| IBIS file stm32wba63_a65_vqfpn68_smps_usb.ibs
[IBIS ver] 4.2
[File name] stm32wba63_a65_vqfpn68_smps_usb.ibs
[File Rev] 2.0
[Date] 17-02-2025
[Source] Data Created at STMicroelectronics
[Notes]  File originated from ELDO simulations.
[Disclaimer]  This information is for modeling purpose only and is
   not guaranted. The information is subject to change without
   notice.
[Copyright] Copyright 2025 STMicroelectronics Inc.
|   Component stm32wba63_a65_vqfpn68_smps_usb
[Component] stm32wba63_a65_vqfpn68_smps_usb
[Manufacturer] STMicroelectronics
[Package]
| variable   typ   min   max
R_pkg  0  NA  NA
L_pkg  0  NA  NA
C_pkg  0  NA  NA
[Pin]   signal_name   model_name
0  VSS  gnd
1  VSSSMPS  nc
2  VDDSMPS  nc
3  VLXSMPS  nc
4  PB12  io8_ft_100m
5  PB11  io8_ft_100m_i2c
6  PA8  io8_ft_100m
7  PA7  io8_ft_100m_i2c_v33
8  PA6  io8_ft_100m_i2c
9  VREFP  nc
10  VDDA  nc
11  PA5  io8_ft_100m
12  PA4  io8_ft_100m_v33
13  PA3  io8_ft_100m
14  PB10  io8_ft_100m_i2c
15  PA2  io8_ft_100m_v33
16  VDD  power
17  PA1  io8_ft_100m
18  PA0  io8_ft_100m
19  PB9  io8_ft_100m
20  VDDUSB  power
21  PD9  io8_ft_100m
22  PD8  io8_ft_100m
23  PD7  io8_ft_100m
24  PD6  io8_ft_100m
25  PD5  io8_ft_100m
26  PB8  io8_ft_100m
27  VDD  power
28  PC15-OSC32_OUT  io_ft_tamp
29  PC14-OSC32_IN  io_ft_tamp
30  PC13  io8_ft_100m_v33
31  VDD  power
32  PB4  io8_ft_100m
33  PE3  io8_ft_100m_hslv
34  PE2  io8_ft_100m_hslv
35  PE1  io8_ft_100m_hslv
36  PE0  io8_ft_100m_hslv
37  PD14  io8_ft_100m_hslv
38  VDD  power
39  PB3  io8_ft_100m_i2c
40  PA15  io8_ft_100m_i2c
41  PA14  io8_ft_100m_v33
42  PA13  io8_ft_100m
43  PA12  io8_ft_100m
44  PA11  io8_ft_100m
45  PB2  io8_ft_100m_i2c_v33
46  PB1  io8_ft_100m_i2c
47  PB0  io8_ft_100m
48  PB15  io8_ft_100m
49  PH3-BOOT0  io8_ft_100m_v33
50  VDD  power
51  NRST  ioreset_v33
52  RF  nc
53  VDDHPA  nc
54  VDDANA  nc
55  VDDRF  nc
56  OSC_OUT  nc
57  OSC_IN  nc
58  VDDRFPA  nc
59  VDD-59  power
60  VDD11  nc
61  PC5  io8_ft_100m
62  PC4  io8_ft_100m
63  PC3  io8_ft_100m
64  PA10  io8_ft_100m
65  PA9  io8_ft_100m
66  PB14  io8_ft_100m_i2c
67  PB13  io8_ft_100m_i2c
68  VDD-68  power
[Package Model]   4b0-vqfn-8x8-68-240827
[Pin Mapping]   pulldown_ref   pullup_ref   | Comment
0  gndio  nc
1  nc  nc
2  nc  nc
3  nc  nc
4  gndio  vddio
5  gndio  vddio
6  gndio  vddio
7  gndio  vddio
8  gndio  vddio
9  nc  nc
10  nc  nc
11  gndio  vddio
12  gndio  vddio
13  gndio  vddio
14  gndio  vddio
15  gndio  vddio
16  nc  vddio
17  gndio  vddio
18  gndio  vddio
19  gndio  vddio
20  nc  vddusb
21  gndio  vddio  | Depending on IO usage
| 21  gndio  vddusb  | Depending on IO usage
22  gndio  vddio  | Depending on IO usage
| 22  gndio  vddusb  | Depending on IO usage
23  gndio  vddio
24  gndio  vddio
25  gndio  vddio
26  gndio  vddio
27  nc  vddio
28  gndio  vddio
29  gndio  vddio
30  gndio  vddio
31  nc  vddio
32  gndio  vddio
33  gndio  vddio
34  gndio  vddio
35  gndio  vddio
36  gndio  vddio
37  gndio  vddio
38  nc  vddio
39  gndio  vddio
40  gndio  vddio
41  gndio  vddio
42  gndio  vddio
43  gndio  vddio
44  gndio  vddio
45  gndio  vddio
46  gndio  vddio
47  gndio  vddio
48  gndio  vddio
49  gndio  vddio
50  nc  vddio
51  gndio  vddio
52  nc  nc
53  nc  nc
54  nc  nc
55  nc  nc
56  nc  nc
57  nc  nc
58  nc  nc
59  nc  vddio
60  nc  nc
61  gndio  vddio
62  gndio  vddio
63  gndio  vddio
64  gndio  vddio
65  gndio  vddio
66  gndio  vddio
67  gndio  vddio
68  nc  vddio
|[Diff Pin]  inv_pin  vdiff  tdelay_typ  tdelay_min  tdelay_max
|24  23  NA  NA  NA  NA
[Model Selector] io8_ft_100m
io8_ft_100m_ls_1v2  "GPIO 100MHz - 5V tolerant - low speed - 1.2V range"
io8_ft_100m_ls_1v8  "GPIO 100MHz - 5V tolerant - low speed - 1.8V range"
io8_ft_100m_ls_3v3  "GPIO 100MHz - 5V tolerant - low speed - 3.3V range"
io8_ft_100m_ms_1v2  "GPIO 100MHz - 5V tolerant - med speed - 1.2V range"
io8_ft_100m_ms_1v8  "GPIO 100MHz - 5V tolerant - med speed - 1.8V range"
io8_ft_100m_ms_3v3  "GPIO 100MHz - 5V tolerant - med speed - 3.3V range"
io8_ft_100m_fs_1v2  "GPIO 100MHz - 5V tolerant - fast speed - 1.2V range"
io8_ft_100m_fs_1v8  "GPIO 100MHz - 5V tolerant - fast speed - 1.8V range"
io8_ft_100m_fs_3v3  "GPIO 100MHz - 5V tolerant - fast speed - 3.3V range"
io8_ft_100m_hs_1v2  "GPIO 100MHz - 5V tolerant - high speed - 1.2V range"
io8_ft_100m_hs_1v8  "GPIO 100MHz - 5V tolerant - high speed - 1.8V range"
io8_ft_100m_hs_3v3  "GPIO 100MHz - 5V tolerant - high speed - 3.3V range"
[Model Selector] io8_ft_100m_hslv
io8_ft_100m_ls_1v2  "GPIO 100MHz - 5V tolerant - low speed - 1.2V range"
io8_ft_100m_ls_1v8  "GPIO 100MHz - 5V tolerant - low speed - 1.8V range"
io8_ft_100m_ls_3v3  "GPIO 100MHz - 5V tolerant - low speed - 3.3V range"
io8_ft_100m_ms_1v2  "GPIO 100MHz - 5V tolerant - med speed - 1.2V range"
io8_ft_100m_ms_1v8  "GPIO 100MHz - 5V tolerant - med speed - 1.8V range"
io8_ft_100m_ms_3v3  "GPIO 100MHz - 5V tolerant - med speed - 3.3V range"
io8_ft_100m_fs_1v2  "GPIO 100MHz - 5V tolerant - fast speed - 1.2V range"
io8_ft_100m_fs_1v8  "GPIO 100MHz - 5V tolerant - fast speed - 1.8V range"
io8_ft_100m_fs_3v3  "GPIO 100MHz - 5V tolerant - fast speed - 3.3V range"
io8_ft_100m_hs_1v2  "GPIO 100MHz - 5V tolerant - high speed - 1.2V range"
io8_ft_100m_hs_1v8  "GPIO 100MHz - 5V tolerant - high speed - 1.8V range"
io8_ft_100m_hs_3v3  "GPIO 100MHz - 5V tolerant - high speed - 3.3V range"
io8_ft_100m_hslv_ls_1v2  "GPIO 100MHz lv opt - 5V tolerant - low speed - 1.2V range"
io8_ft_100m_hslv_ls_1v8  "GPIO 100MHz lv opt - 5V tolerant - low speed - 1.8V range"
io8_ft_100m_hslv_ls_2v5  "GPIO 100MHz lv opt - 5V tolerant - low speed - 2.5V range"
io8_ft_100m_hslv_ms_1v2  "GPIO 100MHz lv opt - 5V tolerant - med speed - 1.2V range"
io8_ft_100m_hslv_ms_1v8  "GPIO 100MHz lv opt - 5V tolerant - med speed - 1.8V range"
io8_ft_100m_hslv_ms_2v5  "GPIO 100MHz lv opt - 5V tolerant - med speed - 2.5V range"
io8_ft_100m_hslv_fs_1v2  "GPIO 100MHz lv opt - 5V tolerant - fast speed - 1.2V range"
io8_ft_100m_hslv_fs_1v8  "GPIO 100MHz lv opt - 5V tolerant - fast speed - 1.8V range"
io8_ft_100m_hslv_fs_2v5  "GPIO 100MHz lv opt - 5V tolerant - fast speed - 2.5V range"
io8_ft_100m_hslv_hs_1v2  "GPIO 100MHz lv opt - 5V tolerant - high speed - 1.2V range"
io8_ft_100m_hslv_hs_1v8  "GPIO 100MHz lv opt - 5V tolerant - high speed - 1.8V range"
io8_ft_100m_hslv_hs_2v5  "GPIO 100MHz lv opt - 5V tolerant - high speed - 2.5V range"
[Model Selector] io8_ft_100m_i2c
io8_ft_100m_ls_1v2  "GPIO 100MHz - 5V tolerant - low speed - 1.2V range"
io8_ft_100m_ls_1v8  "GPIO 100MHz - 5V tolerant - low speed - 1.8V range"
io8_ft_100m_ls_3v3  "GPIO 100MHz - 5V tolerant - low speed - 3.3V range"
io8_ft_100m_ms_1v2  "GPIO 100MHz - 5V tolerant - med speed - 1.2V range"
io8_ft_100m_ms_1v8  "GPIO 100MHz - 5V tolerant - med speed - 1.8V range"
io8_ft_100m_ms_3v3  "GPIO 100MHz - 5V tolerant - med speed - 3.3V range"
io8_ft_100m_fs_1v2  "GPIO 100MHz - 5V tolerant - fast speed - 1.2V range"
io8_ft_100m_fs_1v8  "GPIO 100MHz - 5V tolerant - fast speed - 1.8V range"
io8_ft_100m_fs_3v3  "GPIO 100MHz - 5V tolerant - fast speed - 3.3V range"
io8_ft_100m_hs_1v2  "GPIO 100MHz - 5V tolerant - high speed - 1.2V range"
io8_ft_100m_hs_1v8  "GPIO 100MHz - 5V tolerant - high speed - 1.8V range"
io8_ft_100m_hs_3v3  "GPIO 100MHz - 5V tolerant - high speed - 3.3V range"
io8_ft_100m_i2c_ls_1v2  "GPIO 100MHz with I2C open-drain - 5V tolerant - low speed - 1.2V range"
io8_ft_100m_i2c_ls_1v8  "GPIO 100MHz with I2C open-drain - 5V tolerant - low speed - 1.8V range"
io8_ft_100m_i2c_ls_3v3  "GPIO 100MHz with I2C open-drain - 5V tolerant - low speed - 3.3V range"
io8_ft_100m_i2c_ms_1v2  "GPIO 100MHz with I2C open-drain - 5V tolerant - med speed - 1.2V range"
io8_ft_100m_i2c_ms_1v8  "GPIO 100MHz with I2C open-drain - 5V tolerant - med speed - 1.8V range"
io8_ft_100m_i2c_ms_3v3  "GPIO 100MHz with I2C open-drain - 5V tolerant - med speed - 3.3V range"
io8_ft_100m_i2c_fs_1v2  "GPIO 100MHz with I2C open-drain - 5V tolerant - fast speed - 1.2V range"
io8_ft_100m_i2c_fs_1v8  "GPIO 100MHz with I2C open-drain - 5V tolerant - fast speed - 1.8V range"
io8_ft_100m_i2c_fs_3v3  "GPIO 100MHz with I2C open-drain - 5V tolerant - fast speed - 3.3V range"
io8_ft_100m_i2c_hs_1v2  "GPIO 100MHz with I2C open-drain - 5V tolerant - high speed - 1.2V range"
io8_ft_100m_i2c_hs_1v8  "GPIO 100MHz with I2C open-drain - 5V tolerant - high speed - 1.8V range"
io8_ft_100m_i2c_hs_3v3  "GPIO 100MHz with I2C open-drain - 5V tolerant - high speed - 3.3V range"
io8_ft_100m_i2c_fmp_3v3  "GPIO 100MHz with I2C fm+ open-drain - 5V tolerant - low speed - 3.3V range"
io8_ft_100m_i2c_fmp_1v8  "GPIO 100MHz with I2C fm+ open-drain - 5V tolerant - low speed - 1.8V range"
io8_ft_100m_i2c_fmp_1v2  "GPIO 100MHz with I2C fm+ open-drain - 5V tolerant - low speed - 1.2V range"
[Model Selector] io8_ft_100m_i2c_v33
io8_ft_100m_v33_ls_1v2  "GPIO_V33 100MHz - 5V tolerant - low speed - 1.2V range"
io8_ft_100m_v33_ls_1v8  "GPIO_V33 100MHz - 5V tolerant - low speed - 1.8V range"
io8_ft_100m_v33_ls_3v3  "GPIO_V33 100MHz - 5V tolerant - low speed - 3.3V range"
io8_ft_100m_v33_ms_1v2  "GPIO_V33 100MHz - 5V tolerant - med speed - 1.2V range"
io8_ft_100m_v33_ms_1v8  "GPIO_V33 100MHz - 5V tolerant - med speed - 1.8V range"
io8_ft_100m_v33_ms_3v3  "GPIO_V33 100MHz - 5V tolerant - med speed - 3.3V range"
io8_ft_100m_v33_fs_1v2  "GPIO_V33 100MHz - 5V tolerant - fast speed - 1.2V range"
io8_ft_100m_v33_fs_1v8  "GPIO_V33 100MHz - 5V tolerant - fast speed - 1.8V range"
io8_ft_100m_v33_fs_3v3  "GPIO_V33 100MHz - 5V tolerant - fast speed - 3.3V range"
io8_ft_100m_v33_hs_1v2  "GPIO_V33 100MHz - 5V tolerant - high speed - 1.2V range"
io8_ft_100m_v33_hs_1v8  "GPIO_V33 100MHz - 5V tolerant - high speed - 1.8V range"
io8_ft_100m_v33_hs_3v3  "GPIO_V33 100MHz - 5V tolerant - high speed - 3.3V range"
io8_ft_100m_i2c_v33_ls_1v2  "GPIO_V33 100MHz with I2C open-drain - 5V tolerant - low speed - 1.2V range"
io8_ft_100m_i2c_v33_ls_1v8  "GPIO_V33 100MHz with I2C open-drain - 5V tolerant - low speed - 1.8V range"
io8_ft_100m_i2c_v33_ls_3v3  "GPIO_V33 100MHz with I2C open-drain - 5V tolerant - low speed - 3.3V range"
io8_ft_100m_i2c_v33_ms_1v2  "GPIO_V33 100MHz with I2C open-drain - 5V tolerant - med speed - 1.2V range"
io8_ft_100m_i2c_v33_ms_1v8  "GPIO_V33 100MHz with I2C open-drain - 5V tolerant - med speed - 1.8V range"
io8_ft_100m_i2c_v33_ms_3v3  "GPIO_V33 100MHz with I2C open-drain - 5V tolerant - med speed - 3.3V range"
io8_ft_100m_i2c_v33_fs_1v2  "GPIO_V33 100MHz with I2C open-drain - 5V tolerant - fast speed - 1.2V range"
io8_ft_100m_i2c_v33_fs_1v8  "GPIO_V33 100MHz with I2C open-drain - 5V tolerant - fast speed - 1.8V range"
io8_ft_100m_i2c_v33_fs_3v3  "GPIO_V33 100MHz with I2C open-drain - 5V tolerant - fast speed - 3.3V range"
io8_ft_100m_i2c_v33_hs_1v2  "GPIO_V33 100MHz with I2C open-drain - 5V tolerant - high speed - 1.2V range"
io8_ft_100m_i2c_v33_hs_1v8  "GPIO_V33 100MHz with I2C open-drain - 5V tolerant - high speed - 1.8V range"
io8_ft_100m_i2c_v33_hs_3v3  "GPIO_V33 100MHz with I2C open-drain - 5V tolerant - high speed - 3.3V range"
io8_ft_100m_i2c_fmp_v33_1v2  "GPIO_V33 100MHz with I2C fm+ open-drain - 5V tolerant - low speed - 1.2V range"
io8_ft_100m_i2c_fmp_v33_1v8  "GPIO_V33 100MHz with I2C fm+ open-drain - 5V tolerant - low speed - 1.8V range"
io8_ft_100m_i2c_fmp_v33_3v3  "GPIO_V33 100MHz with I2C fm+ open-drain - 5V tolerant - low speed - 3.3V range"
[Model Selector] io8_ft_100m_v33
io8_ft_100m_v33_ls_1v2  "GPIO_V33 100MHz - 5V tolerant - low speed - 1.2V range"
io8_ft_100m_v33_ls_1v8  "GPIO_V33 100MHz - 5V tolerant - low speed - 1.8V range"
io8_ft_100m_v33_ls_3v3  "GPIO_V33 100MHz - 5V tolerant - low speed - 3.3V range"
io8_ft_100m_v33_ms_1v2  "GPIO_V33 100MHz - 5V tolerant - med speed - 1.2V range"
io8_ft_100m_v33_ms_1v8  "GPIO_V33 100MHz - 5V tolerant - med speed - 1.8V range"
io8_ft_100m_v33_ms_3v3  "GPIO_V33 100MHz - 5V tolerant - med speed - 3.3V range"
io8_ft_100m_v33_fs_1v2  "GPIO_V33 100MHz - 5V tolerant - fast speed - 1.2V range"
io8_ft_100m_v33_fs_1v8  "GPIO_V33 100MHz - 5V tolerant - fast speed - 1.8V range"
io8_ft_100m_v33_fs_3v3  "GPIO_V33 100MHz - 5V tolerant - fast speed - 3.3V range"
io8_ft_100m_v33_hs_1v2  "GPIO_V33 100MHz - 5V tolerant - high speed - 1.2V range"
io8_ft_100m_v33_hs_1v8  "GPIO_V33 100MHz - 5V tolerant - high speed - 1.8V range"
io8_ft_100m_v33_hs_3v3  "GPIO_V33 100MHz - 5V tolerant - high speed - 3.3V range"
[Model Selector] io_ft_tamp
io_ft_tamp_ls_1v2 "io8_ft tamp low speed @ 1.2V"
io_ft_tamp_ls_1v8 "io8_ft tamp low speed @ 1.8V"
io_ft_tamp_ls_3v3 "io8_ft tamp low speed @ 3.3V"
io_ft_tamp_ms_1v2 "io8_ft tamp med speed @ 1.2V"
io_ft_tamp_ms_1v8 "io8_ft tamp med speed @ 1.8V"
io_ft_tamp_ms_3v3 "io8_ft tamp med speed @ 3.3V"
io_ft_tamp_fs_1v2 "io8_ft tamp fast speed @ 1.2V"
io_ft_tamp_fs_1v8 "io8_ft tamp fast speed @ 1.8V"
io_ft_tamp_fs_3v3 "io8_ft tamp fast speed @ 3.3V"
io_ft_tamp_hs_1v2 "io8_ft tamp high speed @ 1.2V"
io_ft_tamp_hs_1v8 "io8_ft tamp high speed @ 1.8V"
io_ft_tamp_hs_3v3 "io8_ft tamp high speed @ 3.3V"
[Model Selector] ioreset_v33
ioreset_v33_1v2 "Reset PAD. 5V tolerant. 1.2V range"
ioreset_v33_1v8 "Reset PAD. 5V tolerant. 1.8V range"
ioreset_v33_3v3 "Reset PAD. 5V tolerant. 3.3V range"
[Define Package Model]  4b0-vqfn-8x8-68-240827
[Manufacturer]  Unknown
[OEM]  Unknown
[Description]  None
[Number Of Pins]  69
[Pin Numbers]
| Pin Num   Terminal Name
52 | RF
51 | NRST
18 | PA0
17 | PA1
15 | PA2
13 | PA3
12 | PA4
11 | PA5
8 | PA6
7 | PA7
6 | PA8
65 | PA9
64 | PA10
44 | PA11
43 | PA12
42 | PA13
41 | PA14
40 | PA15
47 | PB0
46 | PB1
45 | PB2
39 | PB3
32 | PB4
26 | PB8
19 | PB9
14 | PB10
5 | PB11
4 | PB12
67 | PB13
66 | PB14
48 | PB15
63 | PC3
62 | PC4
61 | PC5
30 | PC13
29 | PC14-OSC32_IN
28 | PC15-OSC32_OUT
25 | PD5
24 | PD6
23 | PD7
22 | PD8
21 | PD9
37 | PD14
36 | PE0
35 | PE1
34 | PE2
33 | PE3
49 | PH3-BOOT0
60 | VDD11
16 | VDD
27 | VDD
31 | VDD
38 | VDD
50 | VDD
59 | VDD
68 | VDD
10 | VDDA
54 | VDDANA
53 | VDDHPA
55 | VDDRF
58 | VDDRFPA
2 | VDDSMPS
20 | VDDUSB
3 | VLXSMPS
9 | VREFP
0 | VSS
1 | VSSSMPS
57 | OSC_IN
56 | OSC_OUT
[Model Data]
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[End Model Data]
[End Package Model]
|End [Component]
| Models and submodels in the file (81): io8_ft_100m_fs_1v2 (I/O), io8_ft_100m_fs_1v8 (I/O), io8_ft_100m_fs_3v3 (I/O), io8_ft_100m_hs_1v2 (I/O), io8_ft_100m_hs_1v8 (I/O), io8_ft_100m_hs_3v3 (I/O), io8_ft_100m_hslv_fs_1v2 (I/O), io8_ft_100m_hslv_fs_1v8 (I/O), io8_ft_100m_hslv_fs_2v5 (I/O), io8_ft_100m_hslv_hs_1v2 (I/O), io8_ft_100m_hslv_hs_1v8 (I/O), io8_ft_100m_hslv_hs_2v5 (I/O), io8_ft_100m_hslv_ls_1v2 (I/O), io8_ft_100m_hslv_ls_1v8 (I/O), io8_ft_100m_hslv_ls_2v5 (I/O), io8_ft_100m_hslv_ms_1v2 (I/O), io8_ft_100m_hslv_ms_1v8 (I/O), io8_ft_100m_hslv_ms_2v5 (I/O), io8_ft_100m_i2c_fmp_1v2 (I/O_open_drain), io8_ft_100m_i2c_fmp_1v8 (I/O_open_drain), io8_ft_100m_i2c_fmp_3v3 (I/O_open_drain), io8_ft_100m_i2c_fmp_v33_1v2 (I/O_open_drain), io8_ft_100m_i2c_fmp_v33_1v8 (I/O_open_drain), io8_ft_100m_i2c_fmp_v33_3v3 (I/O_open_drain), io8_ft_100m_i2c_fs_1v2 (I/O_open_drain), io8_ft_100m_i2c_fs_1v8 (I/O_open_drain), io8_ft_100m_i2c_fs_3v3 (I/O_open_drain), io8_ft_100m_i2c_hs_1v2 (I/O_open_drain), io8_ft_100m_i2c_hs_1v8 (I/O_open_drain), io8_ft_100m_i2c_hs_3v3 (I/O_open_drain), io8_ft_100m_i2c_ls_1v2 (I/O_open_drain), io8_ft_100m_i2c_ls_1v8 (I/O_open_drain), io8_ft_100m_i2c_ls_3v3 (I/O_open_drain), io8_ft_100m_i2c_ms_1v2 (I/O_open_drain), io8_ft_100m_i2c_ms_1v8 (I/O_open_drain), io8_ft_100m_i2c_ms_3v3 (I/O_open_drain), io8_ft_100m_i2c_v33_fs_1v2 (I/O_open_drain), io8_ft_100m_i2c_v33_fs_1v8 (I/O_open_drain), io8_ft_100m_i2c_v33_fs_3v3 (I/O_open_drain), io8_ft_100m_i2c_v33_hs_1v2 (I/O_open_drain), io8_ft_100m_i2c_v33_hs_1v8 (I/O_open_drain), io8_ft_100m_i2c_v33_hs_3v3 (I/O_open_drain), io8_ft_100m_i2c_v33_ls_1v2 (I/O_open_drain), io8_ft_100m_i2c_v33_ls_1v8 (I/O_open_drain), io8_ft_100m_i2c_v33_ls_3v3 (I/O_open_drain), io8_ft_100m_i2c_v33_ms_1v2 (I/O_open_drain), io8_ft_100m_i2c_v33_ms_1v8 (I/O_open_drain), io8_ft_100m_i2c_v33_ms_3v3 (I/O_open_drain), io8_ft_100m_ls_1v2 (I/O), io8_ft_100m_ls_1v8 (I/O), io8_ft_100m_ls_3v3 (I/O), io8_ft_100m_ms_1v2 (I/O), io8_ft_100m_ms_1v8 (I/O), io8_ft_100m_ms_3v3 (I/O), io8_ft_100m_v33_fs_1v2 (I/O), io8_ft_100m_v33_fs_1v8 (I/O), io8_ft_100m_v33_fs_3v3 (I/O), io8_ft_100m_v33_hs_1v2 (I/O), io8_ft_100m_v33_hs_1v8 (I/O), io8_ft_100m_v33_hs_3v3 (I/O), io8_ft_100m_v33_ls_1v2 (I/O), io8_ft_100m_v33_ls_1v8 (I/O), io8_ft_100m_v33_ls_3v3 (I/O), io8_ft_100m_v33_ms_1v2 (I/O), io8_ft_100m_v33_ms_1v8 (I/O), io8_ft_100m_v33_ms_3v3 (I/O), io_ft_tamp_fs_1v2 (I/O), io_ft_tamp_fs_1v8 (I/O), io_ft_tamp_fs_3v3 (I/O), io_ft_tamp_hs_1v2 (I/O), io_ft_tamp_hs_1v8 (I/O), io_ft_tamp_hs_3v3 (I/O), io_ft_tamp_ls_1v2 (I/O), io_ft_tamp_ls_1v8 (I/O), io_ft_tamp_ls_3v3 (I/O), io_ft_tamp_ms_1v2 (I/O), io_ft_tamp_ms_1v8 (I/O), io_ft_tamp_ms_3v3 (I/O), ioreset_v33_1v2 (I/O_open_drain), ioreset_v33_1v8 (I/O_open_drain)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
